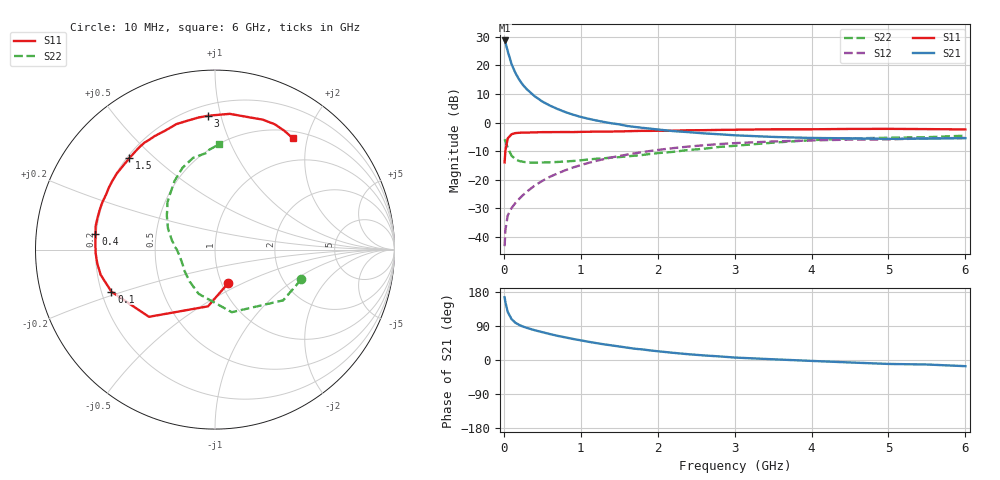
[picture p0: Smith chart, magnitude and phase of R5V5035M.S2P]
! SIEMENS Small Signal Semiconductors
! BFR183
! Si NPN RF Bipolar Junction Transistor in SOT23
! VCE = 0.5 V  IC = 35 mA
! Common Emitter S-Parameters:  May  1996
# GHz  S  MA  R  50
!  f  S11  S21  S12  S22
! GHz  MAG  ANG  MAG  ANG  MAG  ANG  MAG  ANG
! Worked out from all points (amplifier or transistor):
!   36 points, 10 MHz to 6 GHz, reference 50 ohm
!   highest |S21| = 28.8 dB at 10 MHz (marker M1)
!   |S21| within 3 dB of that: start of sweep to 42.99 MHz
!   unconditionally stable (mu >= 1): start of sweep to 26.29 MHz; 115.6 MHz to end of sweep
!   at 250 MHz: K = 1.28, MAG = 16.1 dB, |S12| = -25.4 dB
!   at 1.4 GHz: K = 1.29, MAG = 2.7 dB, |S12| = -12.3 dB
!   at 6 GHz: K = 1.07, MAG = -1.7 dB, |S12| = -5.4 dB
!   S11 on the Smith chart (normalised r, x): 10 MHz: 1.08, -0.42; 100 MHz: 0.24, -0.18; 400 MHz: 0.20, +0.06; 1.5 GHz: 0.21, +0.42; 3 GHz: 0.27, +0.91; 6 GHz: 0.60, +1.76
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0.01  0.1999 -68.1  27.42 165.7  0.0068 68.9  0.5088 -19.0
0.02  0.3184 -97.0  25.48 152.8  0.0129 65.6  0.4734 -36.7
0.05  0.525 -134.5  17.87 127.1  0.0234 53.9  0.3611 -75.0
0.1  0.6229 -157.9  10.62 107.9  0.0316 51.4  0.2628 -110.3
0.15  0.6525 -167.6  7.411 98.4  0.0388 54.8  0.2271 -128.4
0.2  0.6606 -173.4  5.632 92.5  0.0459 58.7  0.2113 -140.0
0.25  0.6651 -178.2  4.527 88.1  0.0536 61.0  0.2052 -148.3
0.3  0.666 178.9  3.813 84.7  0.0615 63.0  0.1997 -153.2
0.4  0.6713 172.7  2.893 78.7  0.0782 65.0  0.1975 -160.9
0.5  0.6778 168.8  2.333 73.5  0.0949 65.8  0.199 -166.9
0.6  0.6784 164.4  1.976 68.4  0.112 65.7  0.2007 -170.6
0.7  0.68 160.1  1.722 63.7  0.1284 64.9  0.2036 -173.5
0.9  0.6799 153.1  1.371 55.5  0.1628 62.9  0.2117 -179.5
1.1  0.6885 145.9  1.163 48.1  0.1959 60.0  0.2248 176.0
1.5  0.6978 133.2  0.928 35.7  0.2591 53.2  0.2472 167.1
2.2  0.7188 112.6  0.707 19.0  0.3553 40.3  0.3057 150.2
3  0.7469 93.0  0.597 6.5  0.4352 25.3  0.3903 130.9
3.5  0.7608 83.8  0.559 1.9  0.4652 16.8  0.4434 120.6
4.5  0.7714 69.8  0.528 -6.5  0.5012 2.8  0.5256 103.4
5  0.7737 64.5  0.517 -10.4  0.5057 -3.5  0.5413 94.7
5.5  0.7662 59.6  0.523 -11.9  0.5271 -7.1  0.5528 94.3
6  0.7568 55.1  0.532 -16.3  0.5355 -13.7  0.588 87.6
